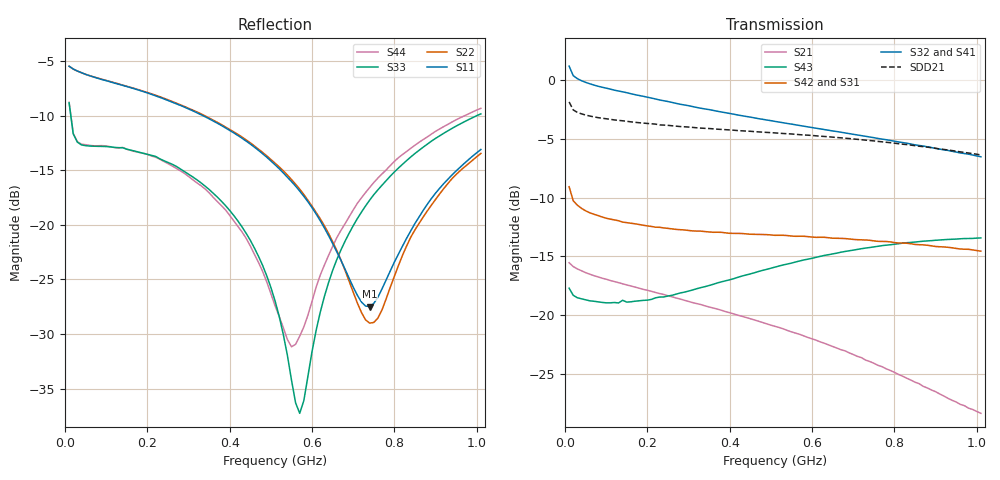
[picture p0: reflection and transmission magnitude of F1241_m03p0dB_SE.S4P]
! Integrated Device Technology
! Corporate Headquarters
! 6024 Silver Creek Valley Road
! San Jose, CA 95138  USA
! Phone:  1-408-284-8200
! Toll Free:  1-800-223-1366
! Webpage:  http://www.idt.com/
! Timing and RF Division
! 515 Groton Road, Suite 102
! Westford, MA 01886-6024
! Device:  F1241
! Description: Dual Intermediate Frequency Digital Variable Gain Amplifier
! Frequency:  10.0 -  500.00 MHz
! Package:  5x5 mm QFN Plastic Package: 32 pin
! Ports:  8 RF, 20 DC
!  Pin  1  = GA3  Pin 17  = RF OUT_B+
!  Pin  2  = GA4  Pin 18  = RF OUT_B-
!  Pin  3  = GA5  Pin 19  = STBY_B
!  Pin  4  = ISET_A  Pin 20  = Ground
!  Pin  5  = ISET_B  Pin 21  = Ground
!  Pin  6  = GB5  Pin 22  = STB_A
!  Pin  7  = GB4  Pin 23  = RF OUT_A-  = Port 4
!  Pin  8  = GB3  Pin 24  = RF OUT_A+  = Port 3
!  Pin  9  = GB2  Pin 25  = NO CONNECT
!  Pin 10  = GB1  Pin 26  = NO CONNECT
!  Pin 11  = RF IN_B+  Pin 27  = VCC
!  Pin 12  = RF IN_B-  Pin 28  = Ground
!  Pin 13  = Ground  Pin 29  = RF IN_A-  = Port 2
!  Pin 14  = VCC  Pin 30  = RF IN_A+  = Port 1
!  Pin 15  = NO CONNECT  Pin 31  = GA1
!  Pin 16  = NO CONNECT  Pin 32  = GA2
! State:  23
! Gain State:  -3.0 dB
! Voltages:  Vcc = +5.00 Volts  Icc approximately 160.0 mA or 80 mA per channel.
! Data:  The device was measured on a custom evaluation board which has
!  individual transmission lines to the RF pins.  Data was collected
!  using a calibrated network analyzer.  The evaluation board was
!  de-embedded using a port reference technique.
!  The reference plane is the edge of the package pin.
!  Only Channel A was measured.
!  This data is in single-ended operation.  If your needs are balanced
!  or differential S-parameters then this file needs to be used a
!  linear simulator.
! Misc:  Lot Code  160028MY
!  Action Tracker AT004
! Date Measured:  2014-08-14
! Date:  2014-08-28  MJV
! Note:
!  Integrated Device Technology supplies this data as a sample of measured
!  data at the package pin for this product.  Your particular data for this
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# Hz S dB R 50
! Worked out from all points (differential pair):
!   101 points, 10 MHz to 1.01 GHz, reference 50 ohm
!   strongest paths, dB at 10 MHz, 260 MHz, 510 MHz, 760 MHz, 1.01 GHz:
!     S32: 1.2, -1.9, -3.5, -5.0, -6.5
!     S41: 1.2, -1.9, -3.6, -5.2, -6.8
!     S42: -9.1, -12.7, -13.2, -13.7, -14.5
!     S31: -9.1, -12.7, -13.3, -13.8, -14.6
!     S43: -17.7, -18.3, -15.9, -14.1, -13.4
!     S21: -15.5, -18.4, -20.9, -24.3, -28.3
!   taken as a pair (ports 2,1 in; 3,4 out), SDD21 dB: -1.9, -3.9, -4.5, -5.2, -6.4
!   lowest |S11| = -27.5 dB at 740 MHz (marker M1), VSWR 1.09, Z = 46.9 - j2.71 ohm
!   |S11| at or under -10 dB: 334.8 MHz to end of sweep
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1e7  -5.48 -7.2  -15.51 -10.7  -34.88 -2.8  -23.69 8.1
     -15.53 -10.7  -5.47 -7.1  -23.71 7.8  -34.95 -3.1
     -9.07 156.5  1.18 168.3  -8.84 -40.8  -17.74 -179.9
     1.23 168.4  -9.07 156.7  -17.70 -179.9  -8.78 -40.6
6e7  -6.35 -10.6  -16.50 -12.8  -35.89 -4.2  -24.04 -4.8
     -16.50 -12.8  -6.34 -10.1  -24.06 -5.1  -35.91 -4.0
     -11.27 151.3  -0.31 164.5  -12.79 -10.3  -18.83 164.1
     -0.28 164.3  -11.28 151.4  -18.77 164.1  -12.73 -10.1
4.2e8  -11.82 -36.8  -19.96 -38.8  -35.38 8.9  -24.72 -19.4
       -19.99 -39.1  -11.72 -33.9  -24.59 -19.2  -35.39 7.0
       -13.12 64.4  -2.98 120.2  -19.65 -19.1  -16.86 103.4
       -3.03 119.0  -13.04 63.8  -16.77 103.2  -20.16 -13.3
5.7e8  -16.91 -51.8  -21.59 -45.8  -34.08 8.9  -24.61 -26.4
       -21.62 -46.2  -16.73 -46.4  -24.30 -26.1  -34.08 6.9
       -13.38 37.7  -3.87 104.7  -37.27 57.6  -15.51 82.3
       -3.98 103.3  -13.28 36.8  -15.38 82.1  -30.20 75.7
6.4e8  -20.98 -65.6  -22.45 -48.5  -33.49 8.0  -24.60 -29.9
       -22.52 -49.0  -20.78 -58.2  -24.20 -29.9  -33.46 5.7
       -13.52 26.8  -4.27 97.7  -25.30 127.2  -15.00 73.1
       -4.42 96.3  -13.41 25.1  -14.85 72.7  -22.81 116.9
7.4e8  -27.49 -137.0  -23.81 -51.1  -32.59 5.1  -24.59 -35.3
       -23.93 -51.4  -29.01 -127.0  -24.10 -35.6  -32.59 2.7
       -13.75 12.5  -4.84 87.9  -17.74 131.2  -14.39 60.4
       -5.04 86.5  -13.62 10.4  -14.24 60.2  -16.58 124.6
1.01e9  -13.10 137.2  -28.17 -45.1  -30.71 -7.3  -24.96 -50.1
        -28.33 -44.0  -13.46 137.9  -24.18 -51.3  -30.63 -10.1
        -14.64 -19.1  -6.52 63.1  -9.84 123.4  -13.60 30.5
        -6.80 62.1  -14.55 -22.3  -13.42 30.5  -9.33 119.6
